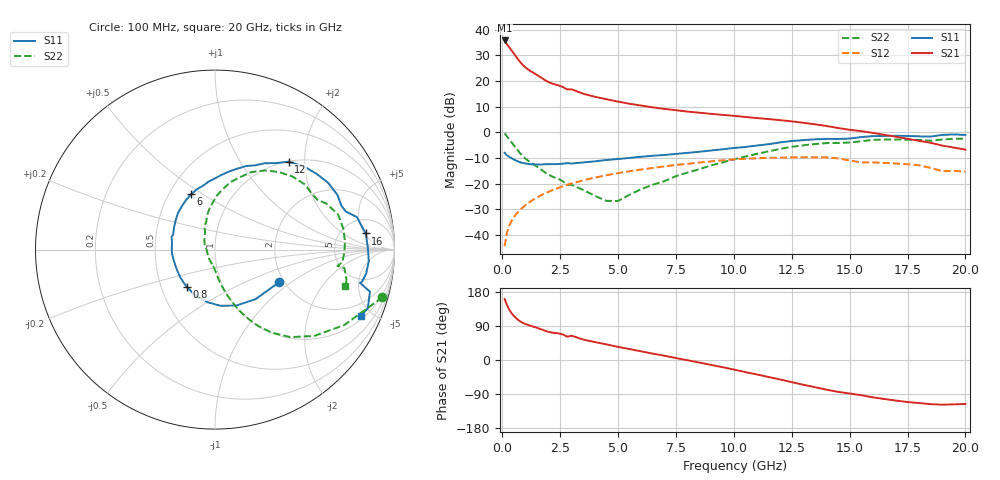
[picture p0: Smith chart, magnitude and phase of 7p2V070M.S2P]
! Infineon Technologies  Discrete & RF Semiconductors
! bfp620
! VCE =  2.0 V,  IC =  70 mA
! Common Emitter S-Parameters:  Sep 2002
# GHz  S  MA  R  50
!  f  S11  S21  S12  S22
! GHz  MAG  ANG  MAG  ANG  MAG  ANG  MAG  ANG
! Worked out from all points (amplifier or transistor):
!   59 points, 100 MHz to 20 GHz, reference 50 ohm
!   highest |S21| = 35.8 dB at 100 MHz (marker M1)
!   |S21| within 3 dB of that: start of sweep to 326.5 MHz
!   unconditionally stable (mu >= 1): 2.154 GHz to 2.242 GHz; 2.596 GHz to 9.863 GHz; 17.18 GHz to end of sweep
!   at 1 GHz: K = 0.88, MSG = 26.8 dB, |S12| = -28.4 dB
!   at 5.5 GHz: K = 1.04, MAG = 11.9 dB, |S12| = -15.1 dB
!   at 20 GHz: K = 1.26, MAG = 1.2 dB, |S12| = -15.2 dB
!   S11 on the Smith chart (normalised r, x): 100 MHz: 1.89, -0.81; 800 MHz: 0.67, -0.30; 6 GHz: 0.64, +0.45; 12 GHz: 1.01, +1.67; 16 GHz: 9, +5; 20 GHz: 1.19, -4.33
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0.1  0.4015 -26.8  61.6 160.9  0.0061 79.4  0.9698 -15.9
0.2  0.357 -50.5  52.1 145.3  0.011 74.3  0.8345 -30.2
0.3  0.3335 -69.2  45.23 133.1  0.0152 71.8  0.7324 -41.1
0.4  0.3143 -84.5  39.4 123.6  0.019 70.1  0.6428 -49.3
0.5  0.2967 -97.5  34.18 116.2  0.0224 69.0  0.5614 -55.6
0.6  0.2814 -108.8  29.61 110.2  0.0257 68.2  0.4894 -60.5
0.7  0.2692 -118.8  25.76 105.2  0.0289 67.6  0.4282 -64.3
0.8  0.26 -127.3  22.65 101.1  0.032 67.1  0.3782 -67.4
0.9  0.2531 -134.5  20.23 97.7  0.0351 66.7  0.3387 -69.8
1.1  0.2441 -145.6  16.95 92.7  0.0414 65.9  0.2837 -73.4
1.9  0.24 -175.6  10.06 76.0  0.0667 61.0  0.1599 -83.8
2.8  0.2523 163.6  6.862 61.5  0.0951 53.6  0.0952 -94.8
3  0.2478 160.1  6.874 64.1  0.1014 51.8  0.0952 -93.5
3.5  0.2603 151.2  5.646 53.7  0.1168 47.1  0.0756 -105.8
6  0.3356 113.5  3.329 22.8  0.1896 22.9  0.0785 139.2
7  0.3632 100.3  2.867 11.3  0.2177 13.2  0.1124 119.5
10.5  0.5208 64.4  1.997 -32.0  0.3067 -26.4  0.3382 82.9
12  0.6395 50.0  1.73 -51.4  0.3205 -44.1  0.4777 64.8
13.5  0.7323 30.4  1.437 -71.7  0.3271 -62.9  0.593 43.4
16  0.8449 6.1  0.979 -98.5  0.2605 -86.9  0.7136 15.9
17  0.8591 -4.3  0.825 -107.1  0.2479 -94.9  0.7256 3.5
20  0.893 -24.3  0.462 -116.0  0.1733 -104.4  0.755 -15.8
